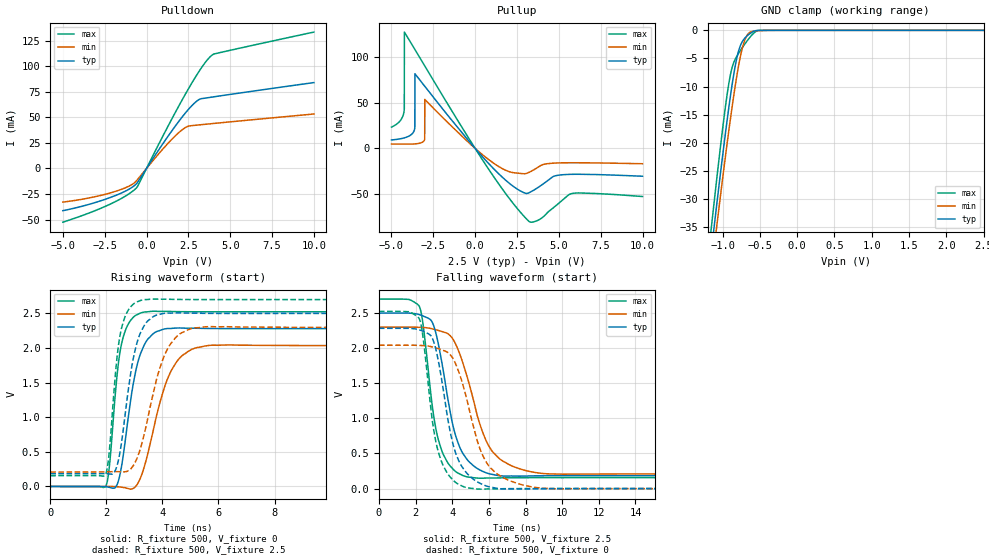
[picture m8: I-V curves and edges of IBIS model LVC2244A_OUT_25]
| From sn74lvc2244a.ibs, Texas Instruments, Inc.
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[Model]   LVC2244A_OUT_25
Model_type  3-state
Enable   Active-Low
Vref =   0
Rref =   500
Cref =   30p
Vmeas =   1.25
| variable   typ   min   max
C_comp   7.02pF   6.59pF   7.42pF
| C_pullup   6.24pF   5.60pF   7.97pF
| C_pulldown   5.64pF   5.20pF   6.41pF
| C_tri-state   7.02pF   6.59pF   7.42pF
[Temperature Range]   40   100   -40
| Ambient temperature   25   85   -40
[Voltage range]   2.5   2.3   2.7
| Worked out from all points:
|   slope of the pulldown table from 0 to 0.375 V, typ, clamps not added: 39.8 ohm
|   slope of the pullup table from 0 to 0.375 V, typ, clamps not added: 47.8 ohm
|   GND clamp passes 1 mA (typ) near -0.67 V on its own axis
|   rising waveform, R_fixture 500, V_fixture 0: 20-80 % time 539ps typ, 826ps min, 364ps max; typ from 0 V to 2.28 V
|   falling waveform, R_fixture 500, V_fixture 2.5: 20-80 % time 1.07ns typ, 1.5ns min, 800ps max; typ from 2.5 V to 0.183 V
|   rising waveform, R_fixture 500, V_fixture 2.5: 20-80 % time 522ps typ, 792ps min, 353ps max; typ from 0.183 V to 2.5 V
|   falling waveform, R_fixture 500, V_fixture 0: 20-80 % time 1.02ns typ, 1.4ns min, 790ps max; typ from 2.28 V to 0 V
[GND Clamp]
| LVC2244A_OUT_25
|   Voltage   I(typ)   I(min)   I(max)
-5V       -524.6mA   -512.3mA   -544.5mA
-1.145V   -38.63mA   -42.25mA   -34.43mA
-1.12V    -35.76mA   -39.47mA   -31.42mA
-1.095V   -32.91mA   -36.71mA   -28.44mA
-1.07V    -30.09mA   -33.97mA   -25.51mA
-955mV    -17.65mA   -21.77mA   -12.96mA
-885mV    -10.83mA   -14.84mA   -7.323mA
-775mV    -3.247mA   -5.592mA   -3.878mA
-710mV    -1.528mA   -2.036mA   -2.596mA
-635mV    -604.2uA   -373uA     -1.27mA
-515mV    -15.29uA   -57.67uA   -13.6uA
2.5V      48.15pA    25.99nA    -1.38nA
[Pulldown]
| LVC2244A_OUT_25
|   Voltage   I(typ)   I(min)   I(max)
-5V       -41.25mA   -32.84mA   -52.5mA
-3.5V     -35.37mA   -29.03mA   -43.95mA
-2.12V    -28.09mA   -23.69mA   -34.47mA
-1.12V    -20.94mA   -17.85mA   -25.55mA
-610mV    -15.04mA   -12.2mA    -19.12mA
1.095V    26.98mA    21.17mA    35.32mA
2.155V    50.78mA    38.1mA     67.73mA
2.515V    57.89mA    41.44mA    78.11mA
3.09V     66.82mA    42.48mA    93.61mA
3.565V    68.89mA    43.26mA    104.7mA
3.915V    69.75mA    43.82mA    110.8mA
10V       83.94mA    53.23mA    133.3mA
[Pullup]
| LVC2244A_OUT_25
|   Voltage   I(typ)   I(min)   I(max)
-5V       9.264mA    4.798mA    23.26mA
-4.25V    11.44mA    4.727mA    40.4mA
-4.235V   11.52mA    4.726mA    43.18mA
-4.23V    11.54mA    4.725mA    126.9mA
-3.615V   21.4mA     4.95mA     108.3mA
-3.605V   22.84mA    4.964mA    108mA
-3.6V     81.41mA    4.971mA    107.8mA
-3.02V    67.99mA    9.735mA    90.18mA
-3.015V   67.88mA    10.18mA    90.03mA
-3.01V    67.76mA    53.49mA    89.87mA
3.235V    -48.18mA   -25.91mA   -79.88mA
10V       -30.3mA    -16.68mA   -52.42mA
[Ramp]
| LVC2244A_OUT_25
| variable   typ   min   max
dV/dt_r   1.39/5.67E-10   1.25/8.69E-10   1.53/3.69E-10
dV/dt_f   1.39/1.09E-09   1.26/1.55E-09   1.53/8.09E-10
R_load = 500
[Rising Waveform]
| LVC2244A_OUT_25
R_fixture =   500
C_fixture =   0
L_fixture =   0
V_fixture =   0
V_fixture_min = 0
V_fixture_max = 0
|   Time   V(typ)   V(min)   V(max)
0s        712.3pV    2.843nV    26.98nV
1.98ns    -3.477mV   -537uV     1.66mV
2.115ns   -13.14mV   -528.4uV   315mV
2.325ns   -13.33mV   -2.68mV    1.358V
2.54ns    285.3mV    -10.54mV   2.056V
2.99ns    1.547V     -20.45mV   2.454V
3.36ns    2.05V      293.8mV    2.52V
4.325ns   2.283V     1.68V      2.527V
5.68ns    2.282V     2.038V     2.523V
50ns      2.281V     2.036V     2.523V
[Falling Waveform]
| LVC2244A_OUT_25
R_fixture =   500
C_fixture =   0
L_fixture =   0
V_fixture =   2.5
V_fixture_min = 2.3
V_fixture_max = 2.7
|   Time   V(typ)   V(min)   V(max)
0s        2.5V       2.3V       2.7V
2.19ns    2.48V      2.297V     2.603V
2.415ns   2.458V     2.295V     2.324V
2.875ns   2.385V     2.278V     1.252V
3.52ns    1.664V     2.231V     482.9mV
4.13ns    803.9mV    2.088V     255.6mV
4.83ns    407.9mV    1.577V     166.2mV
6.18ns    202.4mV    532.8mV    150.8mV
8.805ns   181.7mV    218.8mV    155.4mV
50ns      183.5mV    208.3mV    155.2mV
[Rising Waveform]
| LVC2244A_OUT_25
R_fixture =   500
C_fixture =   0
L_fixture =   0
V_fixture =   2.5
V_fixture_min = 2.3
V_fixture_max = 2.7
|   Time   V(typ)   V(min)   V(max)
0s        183.5mV    208.2mV    155.2mV
1.975ns   185.2mV    210.1mV    172.2mV
2.105ns   180.1mV    211.7mV    505.8mV
2.305ns   219.7mV    213.7mV    1.537V
2.525ns   589.6mV    212.2mV    2.256V
2.95ns    1.825V     293.9mV    2.629V
3.345ns   2.319V     745mV      2.698V
4.205ns   2.505V     2.003V     2.704V
5.52ns    2.501V     2.306V     2.699V
50ns      2.5V       2.3V       2.7V
[Falling Waveform]
| LVC2244A_OUT_25
R_fixture =   500
C_fixture =   0
L_fixture =   0
V_fixture =   0
V_fixture_min = 0
V_fixture_max = 0
|   Time   V(typ)   V(min)   V(max)
0s        2.283V     2.042V     2.524V
2.19ns    2.263V     2.04V      2.425V
2.415ns   2.24V      2.037V     2.139V
2.86ns    2.168V     2.021V     1.081V
3.505ns   1.42V      1.969V     328.5mV
4.095ns   581.9mV    1.827V     107.8mV
4.84ns    206.5mV    1.224V     10.32mV
6.04ns    23.83mV    308.7mV    -4.38mV
8.735ns   -1.822mV   9.784mV    243.6uV
50ns      24.85uV    63.31uV    8.358uV
